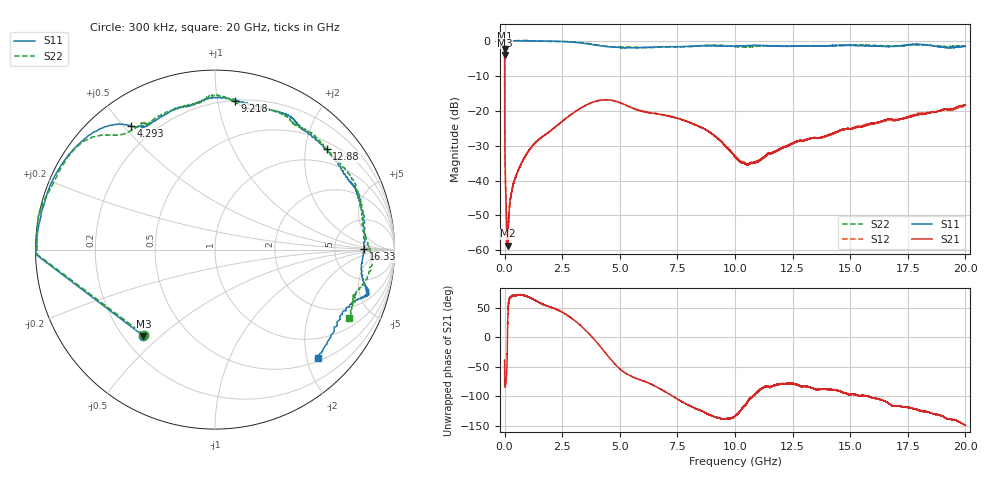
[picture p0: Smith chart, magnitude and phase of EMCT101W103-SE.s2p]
!EMCT101W103
!Johanson Technology Inc.
!www.johansontechnology.com
!Test Board Conditions:
!Substrate Type  RO4350B
!Substrate Thickness  10 mil
!Substrate Dk  3.66
!TL Type: GCPW
!TL Trace Width  22 mil
!TL Gap  14 mil
!PART MODE SINGLE ENDED (AKA BYPASS)
!DUT TOPOLOGY	SERIES-SHUNT
# MHz S  dB  R 50
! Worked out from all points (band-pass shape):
!   20001 points, 300 kHz to 20 GHz, reference 50 ohm
!   highest |S21| = -2.29 dB at 300 kHz (marker M1); lowest = -58.6 dB at 128.3 MHz (marker M2)
!   |S21| within 3 dB of the highest: start of sweep to 636.9 kHz
!   lowest |S11| = -4.1 dB at 300 kHz (marker M3), VSWR 4.33, Z = 13.9 - j22 ohm
!   |S11| at or under -10 dB: nowhere
!   |S22| runs from -4.2 to 0.0 dB; largest |S21 - S12| = 0.0057
!   S11 on the Smith chart (normalised r, x): 300 kHz: 0.28, -0.44; 4.293 GHz: 0.12, +0.53; 9.218 GHz: 0.20, +1.12; 12.88 GHz: 0.65, +2.45; 16.33 GHz: 11, +0; 20 GHz: 0.55, -2.20
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0.3  -4.08 -129.7  -2.29 -38.9  -2.27 -38.8  -4.19 -129.7
101.298  -0.02 179.0  -55.21 -47.5  -54.87 -48.0  -0.08 179.1
128.298  -0.04 178.6  -58.63 11.7  -57.85 10.9  -0.07 178.9
185.297  -0.03 177.9  -50.13 63.4  -50.13 62.3  -0.06 178.1
297.296  -0.04 176.7  -43.43 68.8  -43.40 68.9  -0.06 176.6
436.293  -0.06 175.0  -39.77 70.1  -39.77 69.8  -0.04 174.8
1016.285  -0.09 168.0  -31.79 68.2  -31.78 68.4  -0.01 167.7
2125.268  -0.17 153.5  -25.11 48.9  -25.05 48.7  -0.24 154.5
3334.25  -0.69 132.6  -19.17 18.3  -19.18 18.3  -0.57 138.6
4293.236  -1.60 124.1  -16.95 -22.6  -16.94 -22.7  -1.55 130.3
6667.2  -1.82 106.8  -21.03 -85.6  -20.99 -86.1  -1.91 114.8
9218.162  -1.56 82.4  -27.79 -136.1  -27.80 -135.4  -1.30 88.9
10000.15  -1.60 71.2  -33.17 -134.0  -33.13 -133.6  -1.76 80.1
10829.14  -1.40 62.0  -34.82 -97.9  -34.96 -99.1  -1.68 71.5
12875.11  -1.53 42.1  -28.64 -84.0  -28.55 -83.8  -1.52 52.0
13334.1  -1.59 33.8  -27.85 -86.0  -27.88 -86.0  -1.55 46.3
15168.07  -1.35 19.2  -25.02 -96.6  -24.82 -95.8  -1.30 25.1
16329.06  -1.63 0.1  -23.13 -106.0  -23.26 -107.0  -1.41 13.7
16667.05  -1.71 -5.6  -22.38 -112.0  -22.66 -111.5  -1.55 10.4
18160.03  -1.20 -17.4  -21.02 -125.7  -20.84 -126.0  -1.25 -8.5
19172.01  -1.98 -26.8  -19.59 -137.6  -19.72 -139.1  -1.76 -18.2
20000  -1.58 -46.7  -18.43 -149.2  -18.62 -147.2  -1.55 -27.3
